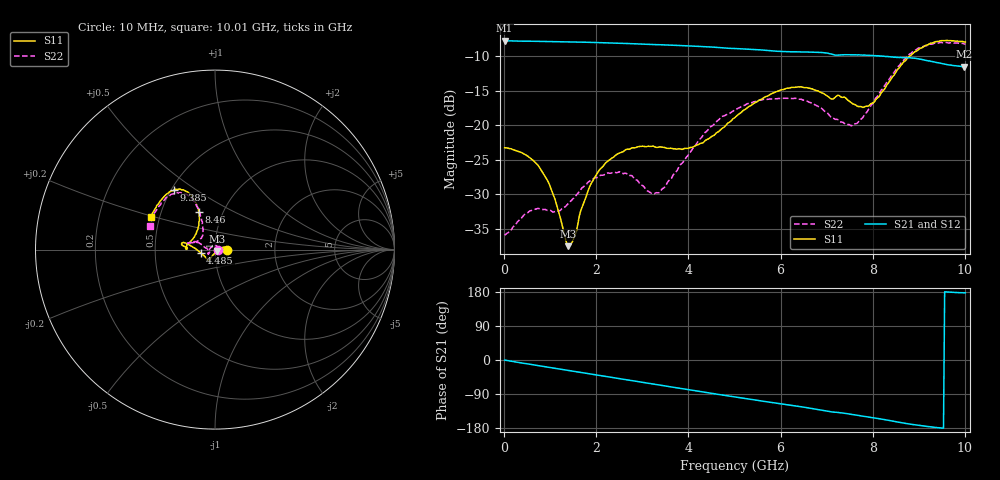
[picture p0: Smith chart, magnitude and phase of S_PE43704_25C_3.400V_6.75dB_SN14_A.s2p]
! Device ID: PE43704
! Dir: z:\PE43704\PE43704_Char_1_20130516\PE43704\AMB\3p400V\6p75dB
! Serial: 14
! Insertion: A
! Impedance: 50 ohm
! Temp: Amb
! VDD: 3.400V
! Attenuation Step: 6.75dB
! IDD: 1.140731e-01mA
#  Hz  S  RI  R  50
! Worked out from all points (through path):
!   401 points, 10 MHz to 10.01 GHz, reference 50 ohm
!   highest |S21| = -7.77 dB at 10 MHz (marker M1); lowest = -11.5 dB at 9.985 GHz (marker M2)
!   group delay of S21, straight-line fit = 52.2 ps
!   lowest |S11| = -37.5 dB at 1.385 GHz (marker M3), VSWR 1.03, Z = 51.1 - j0.822 ohm
!   |S11| at or under -10 dB: start of sweep to 8.799 GHz
!   |S22| runs from -35.9 to -8.0 dB; largest |S21 - S12| = 0.0032
!   S11 on the Smith chart (normalised r, x): 10 MHz: 1.15, +0.00; 4.485 GHz: 0.85, -0.03; 8.46 GHz: 0.77, +0.34; 9.385 GHz: 0.52, +0.41; 10.01 GHz: 0.45, +0.19
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1e7  0.0687 0.000118  0.4086 -0.00161  0.4088 -0.00143  0.016 0.000424
7.85e8  0.0464 0.0139  0.3891 -0.1097  0.3891 -0.1094  0.000752 0.0247
1.06e9  0.031 0.00698  0.3762 -0.1454  0.3761 -0.1453  -0.011 0.0207
1.385e9  0.0106 -0.00804  0.3555 -0.1858  0.3556 -0.1857  -0.0253 0.00931
1.51e9  0.00396 -0.0147  0.3464 -0.2004  0.3465 -0.2002  -0.0295 0.00341
1.685e9  -0.00572 -0.0245  0.3329 -0.2203  0.3329 -0.2202  -0.0346 -0.00524
1.91e9  -0.0153 -0.0357  0.3133 -0.2441  0.3136 -0.244  -0.0374 -0.0145
2.26e9  -0.0248 -0.0494  0.2799 -0.2776  0.28 -0.2773  -0.0387 -0.0231
3.36e9  -0.0389 -0.0576  0.1557 -0.3493  0.156 -0.349  -0.0316 -0.00717
4.035e9  -0.0583 -0.0366  0.0716 -0.3672  0.0719 -0.3672  -0.0611 0.0164
4.485e9  -0.0799 -0.0178  0.015 -0.368  0.0154 -0.3685  -0.0905 0.037
5.01e9  -0.1135 0.00806  -0.0462 -0.3558  -0.0461 -0.3561  -0.1232 0.0385
5.96e9  -0.1727 0.0396  -0.1425 -0.3117  -0.1415 -0.3121  -0.1513 0.0379
6.685e9  -0.1819 0.0231  -0.2085 -0.2658  -0.2084 -0.2658  -0.139 0.0387
7.585e9  -0.1333 0.0488  -0.2632 -0.1885  -0.2629 -0.1881  -0.0732 0.071
7.96e9  -0.1024 0.1001  -0.2811 -0.1527  -0.2814 -0.1534  -0.0679 0.1212
8.36e9  -0.0877 0.187  -0.293 -0.1089  -0.293 -0.1102  -0.0828 0.1996
8.46e9  -0.091 0.2111  -0.2948 -0.0963  -0.2947 -0.0981  -0.0927 0.2216
8.91e9  -0.1397 0.3094  -0.3016 -0.0487  -0.3002 -0.0486  -0.1622 0.3084
9.385e9  -0.2289 0.3319  -0.2844 -0.00902  -0.2846 -0.00813  -0.252 0.3007
9.985e9  -0.3516 0.1902  -0.2644 0.0122  -0.2658 0.0139  -0.3603 0.1417
1.001e10  -0.3571 0.1803  -0.2651 0.0127  -0.267 0.013  -0.3641 0.1329
